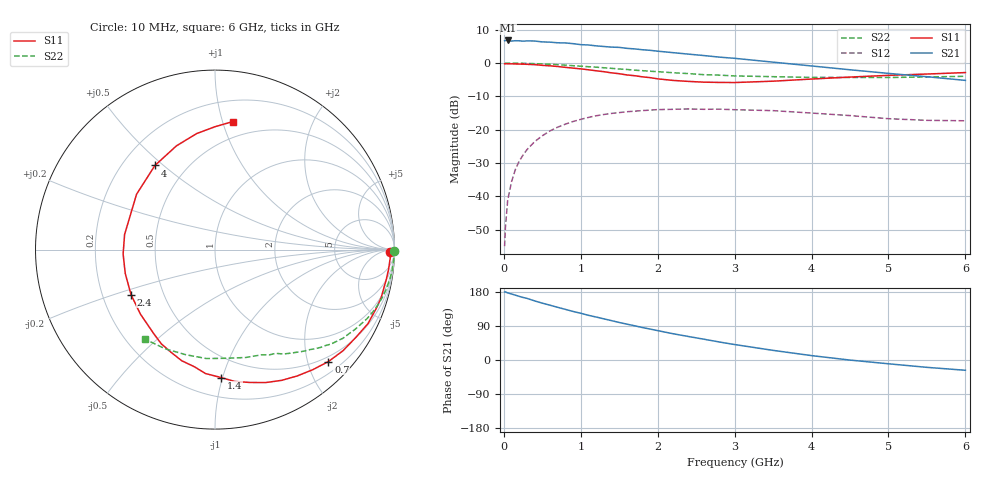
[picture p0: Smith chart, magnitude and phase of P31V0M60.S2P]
! SIEMENS Small Signal Semiconductors
! BFP181
! Si NPN RF Bipolar Junction Transistor in SOT143
! VCE = 1 V  IC = 0.6 mA
! Common Emitter S-Parameters:  March  1996
# GHz  S  MA  R  50
!  f  S11  S21  S12  S22
! GHz  MAG  ANG  MAG  ANG  MAG  ANG  MAG  ANG
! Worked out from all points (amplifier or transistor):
!   36 points, 10 MHz to 6 GHz, reference 50 ohm
!   highest |S21| = 6.8 dB at 50 MHz (marker M1)
!   |S21| within 3 dB of that: start of sweep to 1.918 GHz
!   unconditionally stable (mu >= 1): 3.479 GHz to end of sweep
!   at 250 MHz: K = 0.09, MSG = 17.1 dB, |S12| = -27.6 dB
!   at 1.4 GHz: K = 0.47, MSG = 9.9 dB, |S12| = -15.1 dB
!   at 6 GHz: K = 1.50, MAG = 1.9 dB, |S12| = -17.3 dB
!   S11 on the Smith chart (normalised r, x): 10 MHz: 57, -35; 700 MHz: 0.40, -2.38; 1.4 GHz: 0.34, -0.99; 2.4 GHz: 0.32, -0.23; 4 GHz: 0.33, +0.47; 6 GHz: 0.36, +1.08
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0.01  0.9749 -0.9  2.155 179.7  0.0018 90.0  0.9992 -0.3
0.02  0.9781 -1.0  2.176 179.6  0.0034 90.3  0.9919 -0.6
0.05  0.977 -3.0  2.182 177.1  0.0088 89.0  0.9977 -1.6
0.1  0.9733 -6.6  2.136 174.2  0.0166 85.8  0.9976 -3.2
0.15  0.9689 -9.8  2.162 171.1  0.0254 82.9  0.9947 -4.8
0.25  0.9637 -16.0  2.128 165.0  0.0418 78.7  0.9908 -8.0
0.3  0.9575 -19.5  2.149 162.7  0.0503 76.7  0.9881 -9.6
0.4  0.947 -25.8  2.141 156.0  0.0663 72.0  0.9801 -12.8
0.7  0.8881 -44.6  2.014 139.0  0.1095 59.1  0.9448 -21.7
0.9  0.8401 -56.9  1.954 128.1  0.1331 50.8  0.9127 -27.1
1.1  0.7933 -69.0  1.866 117.9  0.1532 43.3  0.8816 -32.1
1.4  0.7136 -87.3  1.734 103.9  0.1759 33.0  0.8334 -39.2
1.5  0.6926 -94.4  1.718 99.0  0.181 30.0  0.8148 -41.0
1.7  0.6463 -106.7  1.63 90.3  0.19 24.2  0.7824 -45.0
2.2  0.5493 -139.2  1.432 69.3  0.2027 11.7  0.7162 -53.6
2.4  0.5309 -151.8  1.361 62.0  0.2052 7.1  0.6954 -56.8
3  0.5107 170.6  1.178 40.8  0.1998 -4.2  0.6412 -66.1
3.5  0.5349 144.8  1.032 25.4  0.1936 -11.2  0.625 -74.1
4  0.576 125.5  0.905 11.6  0.1781 -16.8  0.6089 -83.9
4.5  0.6166 110.4  0.793 -0.2  0.1632 -21.0  0.6089 -94.5
5.5  0.685 89.9  0.624 -19.4  0.1385 -18.2  0.6183 -116.7
6  0.7201 82.1  0.55 -27.1  0.1364 -15.2  0.6336 -128.1
